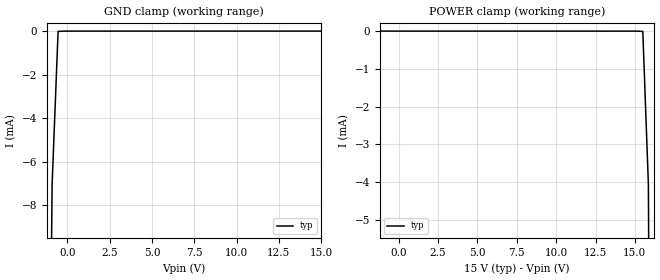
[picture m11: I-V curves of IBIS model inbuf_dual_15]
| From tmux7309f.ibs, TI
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| inbuf_dual_15
[Model]   inbuf_dual_15
Model_type   Input
Vinl = 0.8
Vinh = 1.3
|   typ   min   max
C_comp   1.008417e-12   NA   NA
[Voltage Range]   15   NA   NA
[Temperature Range]   27   NA   NA
[Power Clamp Reference]   15   NA   NA
[GND Clamp Reference]   0   NA   NA
[GND Clamp]
|   Voltage   I(typ)   I(min)   I(max)
-20V      -1.736A    NA         NA
-1.263V   -34.88mA   NA         NA
-909.1mV  -7.032mA   NA         NA
-555.6mV  -13.28uA   NA         NA
15V       953nA      NA         NA
[POWER Clamp]
|   Voltage   I(typ)   I(min)   I(max)
-5V       1.321uA    NA         NA
15.51V    -7.708uA   NA         NA
15.86V    -4.052mA   NA         NA
16.21V    -30.62mA   NA         NA
30V       -1.28A     NA         NA
